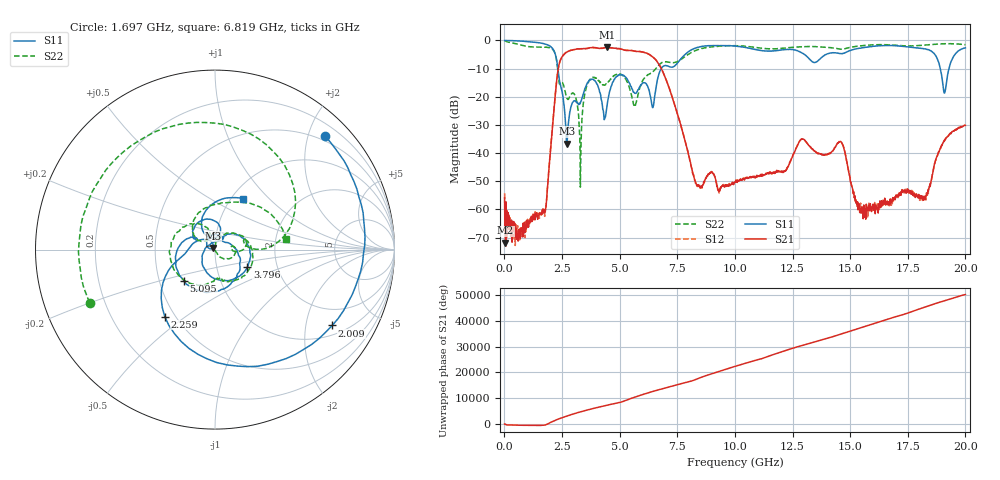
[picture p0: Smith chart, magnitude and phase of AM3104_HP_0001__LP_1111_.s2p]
!Created with skrf (http://scikit-rf.org).
# Hz S RI R 50.0
!freq ReS11 ImS11 ReS21 ImS21 ReS12 ImS12 ReS22 ImS22
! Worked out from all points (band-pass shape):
!   1601 points, 10 MHz to 20 GHz, reference 50 ohm
!   highest |S21| = -2.44 dB at 4.458 GHz (marker M1); lowest = -71.8 dB at 47.48 MHz (marker M2)
!   |S21| within 3 dB of the highest: 2.533 GHz to 6.363 GHz (3.83 GHz wide, 86.1 % of centre)
!   lowest |S11| = -36.6 dB at 2.709 GHz (marker M3), VSWR 1.03, Z = 48.8 + j0.877 ohm
!   |S11| at or under -10 dB: 2.32 GHz to 6.803 GHz (4.483 GHz wide, 98.3 % of centre); 18.91 GHz to 19.29 GHz (379.2 MHz wide, 1.99 % of centre)
!   |S22| runs from -52.1 to -0.1 dB; largest |S21 - S12| = 0.0059
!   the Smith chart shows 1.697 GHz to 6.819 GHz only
!   S11 on the Smith chart (normalised r, x): 1.697 GHz: 0.41, +2.31; 2.009 GHz: 1.32, -2.83; 2.259 GHz: 0.44, -0.42; 3.796 GHz: 1.41, -0.29; 5.095 GHz: 0.67, -0.25; 6.819 GHz: 1.13, +0.71
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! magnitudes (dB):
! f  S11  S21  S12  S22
! 10 MHz  0.0  -55.9  -54.2  -0.1
! 47.48 MHz  0.0  -71.8  -67.8  -0.2
! 1.697 GHz  -1.1  -60.3  -60.0  -2.4
! 2.009 GHz  -2.2  -37.8  -38.0  -2.8
! 2.259 GHz  -6.6  -15.0  -15.0  -6.7
! 2.709 GHz  -36.6  -4.1  -4.1  -20.4
! 3.346 GHz  -21.1  -3.0  -3.0  -31.3
! 3.796 GHz  -13.8  -2.5  -2.5  -13.2
! 4.458 GHz  -23.0  -2.4  -2.4  -15.1
! 5.095 GHz  -12.2  -3.2  -3.2  -12.2
! 5.657 GHz  -18.8  -3.8  -3.8  -23.5
! 6.682 GHz  -12.5  -8.2  -8.2  -8.9
! 6.819 GHz  -9.8  -10.1  -10.2  -7.9
! 8.343 GHz  -2.5  -51.5  -51.5  -3.4
! 10.01 GHz  -2.0  -50.3  -50.3  -1.9
! 13.34 GHz  -7.5  -38.5  -38.4  -2.2
! 14.63 GHz  -4.7  -36.2  -36.3  -3.1
! 15.48 GHz  -2.7  -61.4  -59.6  -1.9
! 16.68 GHz  -1.8  -57.4  -57.4  -1.6
! 18.29 GHz  -3.0  -55.2  -56.7  -1.6
! 19.1 GHz  -18.6  -35.2  -35.3  -1.2
! 20 GHz  -2.6  -30.2  -30.1  -1.5
